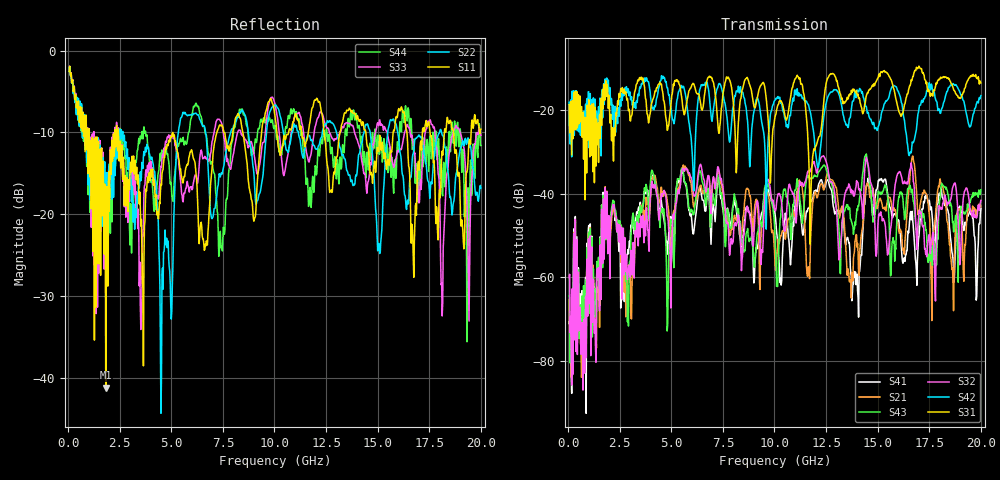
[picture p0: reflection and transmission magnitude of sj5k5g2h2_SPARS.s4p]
! FILE: E:\users\goganessyan\GBX_Backplane\FR408_backplane\1m_OUTBOUND_NEXT\sj5k5g2h2_SPARS.s4p
# MHZ S RI R 50.00
! FREQ  S11  S12  S13  S14
!  S21  S22  S23  S24
!  S31  S32  S33  S34
!  S41  S42  S43  S44
!  REAL  IMAG  REAL  IMAG  REAL  IMAG  REAL  IMAG
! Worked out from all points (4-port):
!   799 points, 50 MHz to 20 GHz, reference 50 ohm
!   strongest paths, dB at 50 MHz, 5.025 GHz, 10.03 GHz, 15.03 GHz, 20 GHz:
!     S31: -18.6, -16.3, -21.6, -12.1, -13.4
!     S42: -18.0, -21.2, -17.6, -23.9, -16.5
!     S32: -60.0, -51.9, -43.9, -46.3, -41.6
!     S43: -64.5, -46.2, -49.4, -39.3, -39.0
!     S21: -65.4, -49.6, -56.6, -42.4, -43.1
!     S41: -71.1, -46.7, -44.7, -36.9, -43.5
!   lowest |S11| = -41.2 dB at 1.825 GHz (marker M1), VSWR 1.02, Z = 50.7 + j0.483 ohm
!   |S11| at or under -10 dB: 1.027 GHz to 2.272 GHz (1.245 GHz wide, 75.5 % of centre); 2.434 GHz to 7.206 GHz (4.772 GHz wide, 99 % of centre); 14.43 GHz to 15.75 GHz (1.323 GHz wide, 8.77 % of centre)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
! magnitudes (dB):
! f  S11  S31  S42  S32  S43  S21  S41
! 50 MHz  -2.5  -18.6  -18.0  -60.0  -64.5  -65.4  -71.1
! 1.825 GHz  -41.2  -12.8  -16.7  -50.7  -51.0  -48.4  -49.6
! 11.15 GHz  -8.4  -11.9  -16.6  -39.7  -38.5  -38.3  -41.0
! 11.75 GHz  -8.2  -44.2  -20.7  -34.1  -36.2  -50.8  -41.9
! 12.72 GHz  -17.1  -11.2  -15.6  -37.1  -37.2  -36.6  -38.8
! 13.65 GHz  -7.1  -16.0  -21.8  -38.1  -43.5  -61.2  -53.5
! 20 GHz  -9.6  -13.4  -16.5  -41.6  -39.0  -43.1  -43.5
